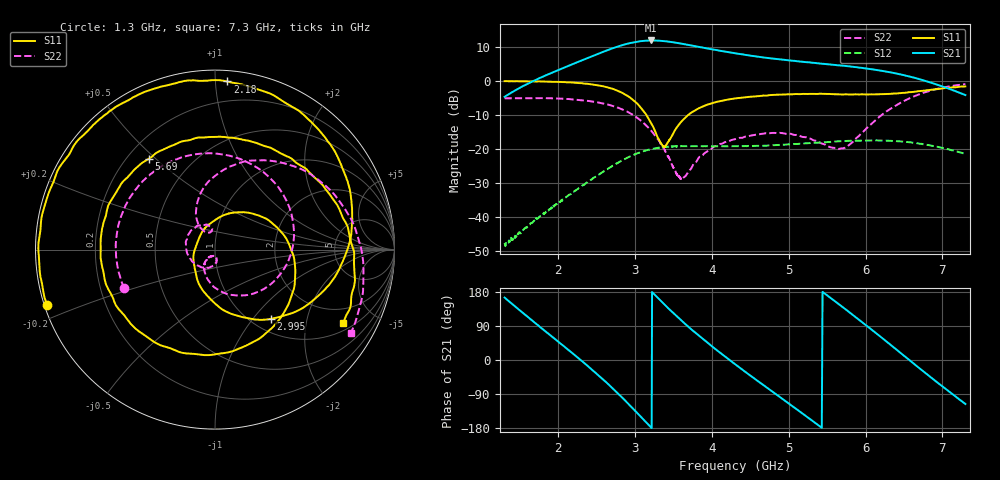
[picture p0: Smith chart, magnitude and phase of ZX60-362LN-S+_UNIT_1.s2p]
!Mini-Circuits Laboratory
!Date: 12/20/2011 at 1:34:49 PM
!Model: ZX60-362LN-S+
!AP#111506
!Run / Lot / Date Code: MFX1750 / N/A / 0949
!Fixture: N/A
!Connection: PORT 1-INPUT; PORT 2-OUTPUT
!S/N: Unit# 1
!Vcc=5V, Icc=18.19mA.
!Network Analyzer: PNA-X N5242A - 423 4 ports;  Serial number: 74302
# Hz  S  dB  R  50
!Frequency  S11 dB  S11 Deg  S21 dB  S21 Deg  S12 dB  S12 Deg  S22 dB  S22 Deg
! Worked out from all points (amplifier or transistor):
!   1000 points, 1.3 GHz to 7.3 GHz, reference 50 ohm
!   highest |S21| = 11.8 dB at 3.205 GHz (marker M1)
!   |S21| within 3 dB of that: 2.624 GHz to 4.095 GHz (1.471 GHz wide, 43.8 % of centre)
!   unconditionally stable (mu >= 1): start of sweep to end of sweep
!   at 2.47 GHz: K = 1.48, MAG = 13.9 dB, |S12| = -28.4 dB
!   at 3.471 GHz: K = 1.42, MAG = 11.5 dB, |S12| = -19.4 dB
!   at 7.3 GHz: K = 1.30, MAG = 5.4 dB, |S12| = -21.6 dB
!   S11 on the Smith chart (normalised r, x): 1.3 GHz: 0.01, -0.16; 2.18 GHz: 0.07, +1.07; 2.995 GHz: 1.21, -1.23; 5.69 GHz: 0.29, +0.48; 7.3 GHz: 1.28, -3.28
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1.3e9  -0.14 -161.6  -4.76 164.8  -47.75 95.9  -5.18 -157.0
1.835e9  -0.26 131.2  1.57 75.1  -38.77 36.5  -5.13 134.5
2.18e9  -0.55 85.8  4.83 18.3  -32.94 -8.6  -5.49 85.1
2.3e9  -0.73 69.2  5.95 -1.7  -31.13 -26.5  -5.73 66.7
2.5e9  -1.28 39.3  7.77 -36.3  -28.00 -56.1  -6.33 34.4
2.63e9  -1.91 18.6  8.90 -60.0  -26.07 -77.6  -6.93 11.8
2.83e9  -3.54 -17.3  10.45 -99.0  -23.43 -113.0  -8.44 -25.5
2.995e9  -6.10 -51.3  11.36 -133.1  -21.67 -144.7  -10.41 -57.8
3.205e9  -12.40 -105.8  11.85 -177.5  -20.16 174.0  -14.64 -98.8
3.3e9  -17.00 -146.2  11.78 162.7  -19.76 155.1  -17.34 -115.2
3.488e9  -15.88 91.7  11.33 125.3  -19.36 120.0  -25.13 -128.6
3.68e9  -10.31 39.0  10.59 90.0  -19.26 86.5  -27.28 -82.1
3.99e9  -6.70 -14.5  9.30 37.7  -19.31 37.1  -20.12 -104.1
4.3e9  -5.24 -59.7  8.09 -10.9  -19.25 -8.3  -17.25 -145.3
4.54e9  -4.63 -92.0  7.27 -47.1  -19.21 -42.8  -16.03 -176.5
4.77e9  -4.22 -122.2  6.56 -81.0  -19.05 -74.6  -15.40 155.0
5.3e9  -3.88 170.8  5.29 -159.3  -18.35 -148.7  -17.28 104.3
5.69e9  -4.06 126.1  4.46 141.5  -17.80 154.8  -19.92 109.7
5.99e9  -4.04 95.1  3.65 94.3  -17.61 109.6  -14.57 121.9
6.3e9  -3.91 65.8  2.56 44.2  -17.68 61.6  -8.63 97.2
6.82e9  -2.75 18.1  -0.34 -40.8  -18.95 -20.0  -3.09 32.5
7.3e9  -1.69 -29.9  -4.24 -116.0  -21.56 -91.8  -1.03 -31.4
